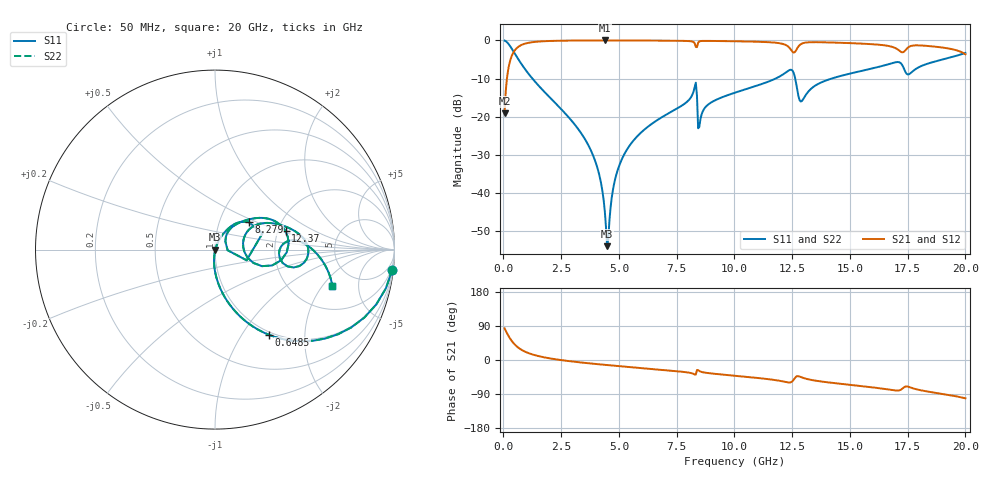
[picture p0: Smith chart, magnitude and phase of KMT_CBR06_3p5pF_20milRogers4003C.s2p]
! Data measured by Modelithics Inc. support@modelithics.com 813-866-6335
! KEMET CBR0603 3.5pF, Pad Width= 0.851mm, Pad Length= 0.64mm, Pad Gap= 0.62mm, 20mil Rogers 4003C substrate Data, January 2022
# hz S ma R 50
! 2 Port Network Data from SP1.SP block
! freq  magS11  angS11  magS21  angS21  magS12  angS12  magS22  angS22
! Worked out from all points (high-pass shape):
!   401 points, 50 MHz to 20 GHz, reference 50 ohm
!   highest |S21| = -0.02 dB at 4.389 GHz (marker M1); lowest = -19.2 dB at 50 MHz (marker M2)
!   |S21| within 3 dB of the highest: 446.9 MHz to 12.52 GHz (12.08 GHz wide, 186 % of centre); 12.62 GHz to 17.22 GHz (4.598 GHz wide, 30.8 % of centre)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
!   lowest |S11| = -54.0 dB at 4.489 GHz (marker M3), VSWR 1.00, Z = 50.2 - j0.113 ohm
!   |S11| at or under -10 dB: 1.252 GHz to 11.79 GHz (10.53 GHz wide, 162 % of centre); 12.63 GHz to 14.21 GHz (1.581 GHz wide, 11.8 % of centre)
!   |S22| runs from -54.0 to -0.1 dB; largest |S21 - S12| = 0
!   S11 on the Smith chart (normalised r, x): 50 MHz: 1, -18; 648.5 MHz: 0.96, -1.33; 8.279 GHz: 1.38, +0.45; 12.37 GHz: 2.21, +0.54; 20 GHz: 3.29, -2.52
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5e7  0.9939 -6.5  0.1102 83.5  0.1102 83.5  0.9939 -6.5
2.99375e8  0.8318 -34.6  0.5544 55.4  0.5544 55.4  0.8318 -34.6
6.485e8  0.5629 -57.6  0.8256 32.3  0.8256 32.3  0.5629 -57.6
1.4465e9  0.2703 -78.4  0.9616 11.4  0.9616 11.4  0.2703 -78.4
3.391625e9  0.059 -95.2  0.9965 -6.7  0.9965 -6.7  0.059 -95.2
4.089875e9  0.02018 -96.0  0.9979 -11.1  0.9979 -11.1  0.02018 -96.0
4.389125e9  0.005722 -83.9  0.998 -12.8  0.998 -12.8  0.005722 -83.9
4.488875e9  0.002006 -34.0  0.998 -13.3  0.998 -13.3  0.002006 -34.0
4.838e9  0.01527 67.4  0.9978 -15.3  0.9978 -15.3  0.01527 67.4
5.13725e9  0.0282 69.0  0.9974 -16.9  0.9974 -16.9  0.0282 69.0
6.73325e9  0.09321 63.1  0.9929 -25.4  0.9929 -25.4  0.09321 63.1
8.279375e9  0.2431 39.1  0.9181 -38.3  0.9181 -38.3  0.2431 39.1
8.52875e9  0.09268 49.2  0.979 -30.5  0.979 -30.5  0.09268 49.2
8.877875e9  0.1455 53.6  0.9845 -34.7  0.9845 -34.7  0.1455 53.6
1.0025e10  0.2065 47.3  0.9742 -41.6  0.9742 -41.6  0.2065 47.3
1.236912e10  0.4061 14.5  0.8076 -59.4  0.8076 -59.4  0.4061 14.5
1.26185e10  0.33 -15.5  0.7033 -47.1  0.7033 -47.1  0.33 -15.5
1.286788e10  0.1579 4.5  0.8892 -44.7  0.8892 -44.7  0.1579 4.5
1.336662e10  0.239 31.3  0.9472 -53.1  0.9472 -53.1  0.239 31.3
1.670825e10  0.4907 8.3  0.8409 -78.2  0.8409 -78.2  0.4907 8.3
1.755612e10  0.3597 -0.2  0.8225 -71.1  0.8225 -71.1  0.3597 -0.2
2e10  0.6844 -17.3  0.6575 -101.1  0.6575 -101.1  0.6844 -17.3
